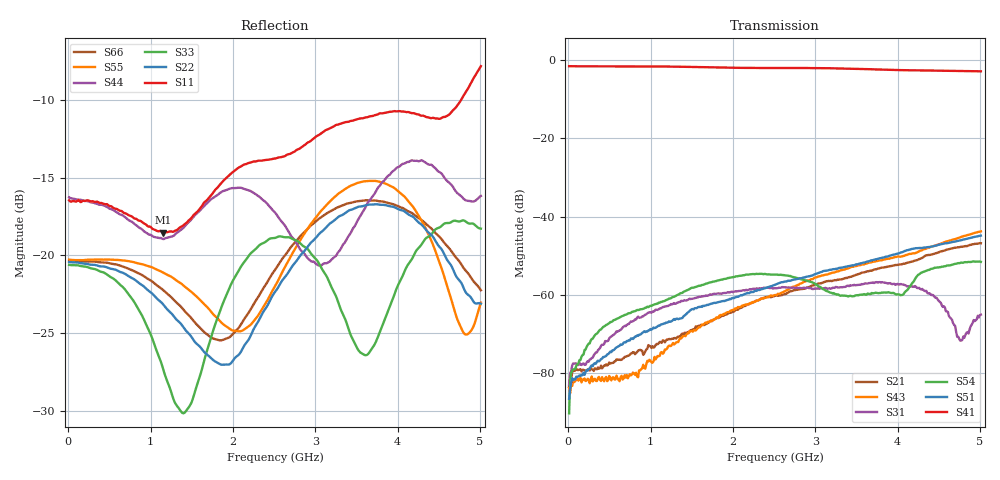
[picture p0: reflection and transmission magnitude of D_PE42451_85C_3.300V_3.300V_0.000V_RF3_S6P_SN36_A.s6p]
! Device ID: PE42451
! Serial: 36
! Insertion: A
! Temp: 85C
! VDD: 3.300
! Control_Hi: 100.000
! Control_Lo: 0.000
! Logic State: RF3
! Port 1: RFC
! Port 2: RF1
! Port 3: RF2
! Port 4: RF3
! Port 5: RF4
! Port 6: RF5
! V1 = 3.30
! V2 = 3.30
! V3 = 0.00
! V4 = 0.00
! IDD: 1.701480e-05
#  Hz  S  RI  R  50
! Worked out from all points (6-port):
!   401 points, 10 MHz to 5.01 GHz, reference 50 ohm
!   strongest paths, dB at 10 MHz, 1.26 GHz, 2.51 GHz, 3.76 GHz, 5.01 GHz:
!     S41: -1.6, -1.7, -2.0, -2.4, -2.9
!     S51: -86.5, -66.6, -57.4, -50.7, -44.8
!     S54: -90.2, -60.6, -54.8, -59.5, -51.5
!     S31: -82.9, -62.4, -58.2, -56.8, -65.0
!     S43: -83.7, -72.6, -60.0, -51.3, -43.7
!     S21: -83.4, -71.1, -60.2, -53.2, -46.8
!   lowest |S11| = -18.5 dB at 1.147 GHz (marker M1), VSWR 1.27, Z = 57.3 - j10.4 ohm
!   |S11| at or under -10 dB: start of sweep to 4.767 GHz
